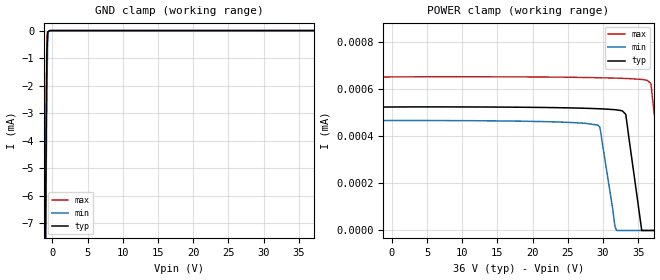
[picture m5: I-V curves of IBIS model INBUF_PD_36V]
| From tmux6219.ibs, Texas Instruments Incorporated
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| Model5
[Model]   INBUF_PD_36V
Model_type   Input
Vinl = 0.8
Vinh = 1.3
|   typ   min   max
C_comp   1.85pF   1.7pF   2.1pF
[Voltage Range]   36   32.4   39.6
[Temperature Range]   27   130   -40
[Power Clamp Reference]   36   32.4   39.6
[GND Clamp Reference]   0   0   0
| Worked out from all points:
|   GND clamp passes 1 mA (typ) near -0.80 V on its own axis
[GND Clamp]
|   Voltage   I(typ)   I(min)   I(max)
-36V      -1.895A    -1.893A    -1.898A
-1.116V   -13.43mA   -14.99mA   -12.38mA
-1.008V   -8.362mA   -10.05mA   -7.209mA
-900mV    -3.84mA    -5.586mA   -2.655mA
-792mV    -816uA     -2.162mA   -233.7uA
-684mV    -53.99uA   -416.1uA   -43.54uA
-576mV    -36.09uA   -34.92uA   -29.16uA
-360mV    -303.8nA   -847.4nA   -394.2nA
72V       0A         0A         0A
[POWER Clamp]
|   Voltage   I(typ)   I(min)   I(max)
-36V      672.7uA    265.8uA    1.426mA
-22.18V   142uA      1.548uA    499uA
-19.69V   41.59uA    450.1nA    306uA
-18.5V    989.5nA    454.1nA    213.4uA
-18.29V   496.1nA    454.9nA    196.5uA
-15.7V    510.8nA    459.6nA    3.609uA
-15.48V   511.3nA    459.8nA    647.8nA
29.23V    516.9nA    447.5nA    648.5nA
32.69V    508.2nA    0A         645.7nA
36.25V    0A         0A         637.2nA
39.38V    0A         0A         0A
72V       0A         0A         0A
